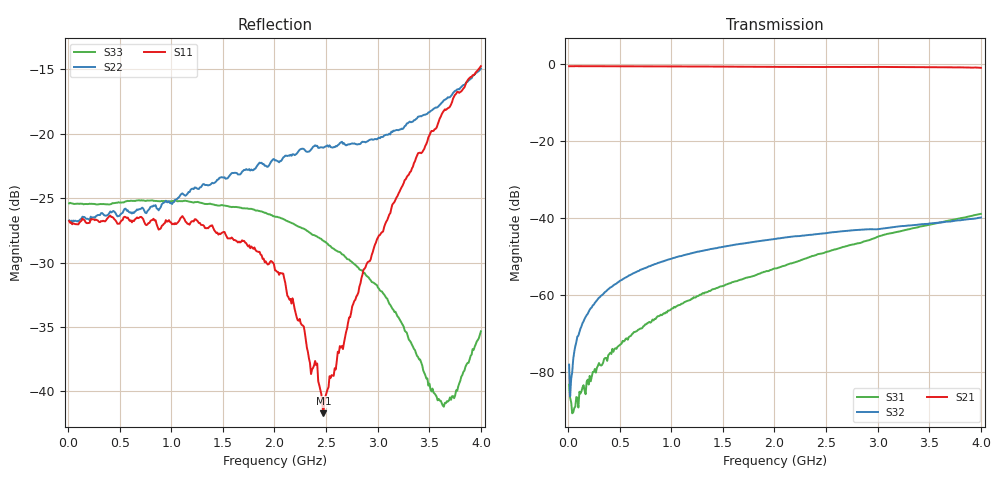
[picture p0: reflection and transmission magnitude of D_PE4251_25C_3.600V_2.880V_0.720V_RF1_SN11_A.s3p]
! Device ID: PE4251_SoldCshunt_081809
! Dir: c:\Test Bench Repositories\Bench_Software_CVI_Version_8\trunk\PSC 4Port_VNA Bench\datalog\4250\TEST\PE4251_SoldCshunt_081809\25C\3p600000\RF1
! Serial: 11
! Insertion: A
! Temp: 25C
! VDD: 3.600
! Control_Hi: 80.000
! Control_Lo: 20.000
! Logic State: RF1
! Port 1: RFC
! Port 2: RF1
! Port 3: RF2
! V1 = 0.72
! V2 = 2.88
! V3 = 0.72
! IDD: 5.388700e-05
! FILE NAME
! DATE 08/18/09  20:13
! CORRECTED  DATA
#  Hz  S  RI  R  50.00
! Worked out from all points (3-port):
!   401 points, 10 MHz to 4 GHz, reference 50 ohm
!   strongest paths, dB at 10 MHz, 1.008 GHz, 2.005 GHz, 3.002 GHz, 4 GHz:
!     S21: -0.6, -0.6, -0.7, -0.7, -1.0
!     S32: -78.2, -50.6, -45.5, -43.0, -39.9
!     S31: -83.4, -63.6, -53.2, -44.9, -39.0
!   lowest |S11| = -41.7 dB at 2.474 GHz (marker M1), VSWR 1.02, Z = 50 - j0.82 ohm
!   |S11| at or under -10 dB: start of sweep to end of sweep
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1e7  0.0458 1.06e-05  0.9374 -0.00371  2.81e-05 -5e-05
     0.938 -0.00399  0.0461 4.06e-05  0.0001 -8.66e-05
     3.05e-05 -5.99e-05  9.85e-05 7.37e-05  0.0537 -0.000235
3.9925e7  0.0445 -0.00022  0.9394 -0.0153  2.82e-05 -1.77e-05
          0.9394 -0.0152  0.0454 -0.000311  3.16e-05 0.000116
          2.58e-05 -1.24e-05  2.82e-05 9.36e-05  0.0537 -0.000414
1.99525e8  0.0451 -0.000624  0.9364 -0.068  -7.9e-08 -7.88e-05
           0.9356 -0.0683  0.0466 -0.000888  5.85e-05 0.000606
           4.01e-06 -6.76e-05  5.87e-05 0.000595  0.0534 -0.00136
5.18725e8  0.0459 -0.00402  0.9214 -0.1709  -0.000157 -0.00018
           0.9208 -0.1708  0.049 -0.00285  0.000164 0.00155
           -0.000152 -0.000174  0.000153 0.00155  0.0539 -0.00484
1.137175e9  0.0429 -0.0157  0.8585 -0.3629  -0.00077 -0.000252
            0.8587 -0.3619  0.0549 -0.0173  0.000577 0.00325
            -0.000773 -0.000243  0.000592 0.00326  0.0546 -0.00661
2.005e9  0.0266 -0.0129  0.7153 -0.5809  -0.00219 -0.000147
         0.7148 -0.5811  0.0687 -0.0387  0.00112 0.00519
         -0.00219 -0.000162  0.00112 0.0052  0.0475 -0.00437
2.473825e9  -0.000431 -0.0082  0.6203 -0.6771  -0.00348 -0.000156
            0.6177 -0.6759  0.063 -0.0619  0.00124 0.00613
            -0.00347 -0.000147  0.00124 0.00615  0.0385 -0.000501
2.872825e9  -0.02 -0.0223  0.5268 -0.7523  -0.00495 4.5e-05
            0.5286 -0.7504  0.0423 -0.0829  0.00129 0.0069
            -0.00495 3.1e-05  0.00132 0.00693  0.0287 0.00233
3.62095e9  -0.0997 -0.0655  0.3105 -0.8545  -0.00859 0.00174
           0.312 -0.8551  -0.047 -0.1235  0.000345 0.00872
           -0.00861 0.00172  0.000363 0.00871  0.00238 0.00868
4e9  -0.1648 -0.0799  0.1771 -0.8803  -0.0108 0.00315
     0.1761 -0.8774  -0.127 -0.1266  -0.000327 0.0101
     -0.0108 0.00313  -0.000343 0.0101  -0.0137 0.0103
